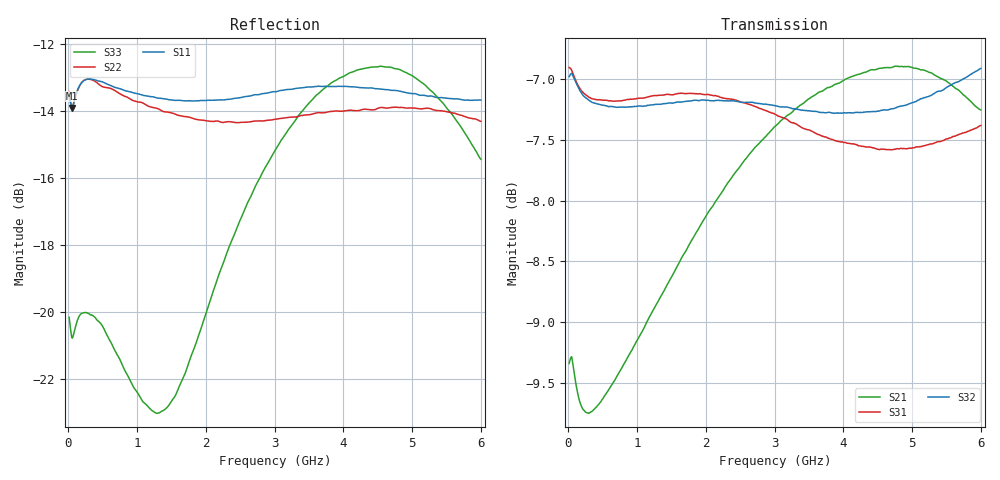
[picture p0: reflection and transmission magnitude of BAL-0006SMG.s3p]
! MARKI MICROWAVE INC.
! Email:  info@markimicrowave.com  Phone:  408-778-4200
! Model Number:  BAL-0006SM  Date:  12/12
! Filename:		BAL-0006SM.S3P  Version: 1.0
! Description:  3-port S-parameter data for Balun BAL-0006SM
! Frequency Range: 	10 MHz to 6 GHz
! Port Configuration:	PORT 1: OUTPUT (0 DEGREE), PORT 2: OUTPUT (180 DEGREE), PORT 3:COMMON
! S3P File: Measurements: Mag<S11> Ang<S11> Mag<S12> Ang<S12> Mag<S13> Ang<S13>! row 1
!  Mag<S21> Ang<S21> Mag<S22> Ang<S22> Mag<S23> Ang<S23>! row 2
!  Mag<S31> Ang<S31> Mag<S32> Ang<S32> Mag<S33> Ang<S33>! row 3
# Hz S  dB  R 50
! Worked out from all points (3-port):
!   801 points, 10 MHz to 6 GHz, reference 50 ohm
!   strongest paths, dB at 10 MHz, 1.508 GHz, 3.005 GHz, 4.503 GHz, 6 GHz:
!     S32: -7.0, -7.2, -7.2, -7.3, -6.9
!     S31: -6.9, -7.1, -7.3, -7.6, -7.4
!     S21: -9.3, -8.6, -7.4, -6.9, -7.3
!   lowest |S11| = -13.9 dB at 47.44 MHz (marker M1), VSWR 1.50, Z = 33.3 + j1.51 ohm
!   |S11| at or under -10 dB: start of sweep to end of sweep
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1e7  -13.56 166.4  -9.33 5.0  -6.90 -0.7
     -9.34 4.4  -13.43 165.5  -6.95 179.7
     -6.91 0.2  -6.98 -179.0  -20.15 165.0
4.74375e7  -13.92 173.8  -9.30 -2.5  -6.92 -4.2
           -9.28 -2.5  -13.90 173.2  -6.93 175.9
           -6.93 -4.4  -6.95 175.7  -20.75 173.4
9.609125e8  -13.47 104.6  -9.19 -65.7  -7.16 -86.0
            -9.19 -65.7  -13.71 101.5  -7.21 92.5
            -7.16 -85.8  -7.23 92.6  -22.28 126.1
1.851925e9  -13.70 39.8  -8.27 -131.7  -7.12 -166.0
            -8.27 -131.6  -14.25 35.4  -7.17 11.7
            -7.12 -165.9  -7.18 11.8  -20.95 107.6
2.361075e9  -13.65 4.4  -7.83 -171.0  -7.17 147.9
            -7.82 -170.9  -14.33 -0.3  -7.17 -34.5
            -7.17 148.1  -7.18 -34.5  -17.94 79.5
3.005e9  -13.43 -39.5  -7.40 138.2  -7.28 89.8
         -7.39 138.3  -14.25 -43.3  -7.20 -92.8
         -7.29 89.9  -7.22 -92.7  -15.18 30.7
3.858575e9  -13.28 -93.3  -7.06 70.0  -7.49 13.4
            -7.05 70.1  -14.01 -95.2  -7.26 -169.4
            -7.50 13.7  -7.28 -169.1  -13.12 -39.9
4.644762e9  -13.37 -139.4  -6.92 6.6  -7.58 -56.5
            -6.91 6.7  -13.92 -140.1  -7.24 121.0
            -7.58 -56.2  -7.26 121.1  -12.70 -104.9
5.266225e9  -13.56 -172.6  -6.97 -44.0  -7.53 -111.8
            -6.95 -43.9  -13.94 -173.5  -7.11 66.0
            -7.53 -111.5  -7.14 66.2  -13.39 -152.6
6e9  -13.68 151.6  -7.28 -102.8  -7.38 -177.4
     -7.26 -102.7  -14.31 148.6  -6.89 1.2
     -7.38 -177.0  -6.91 1.4  -15.44 160.1
